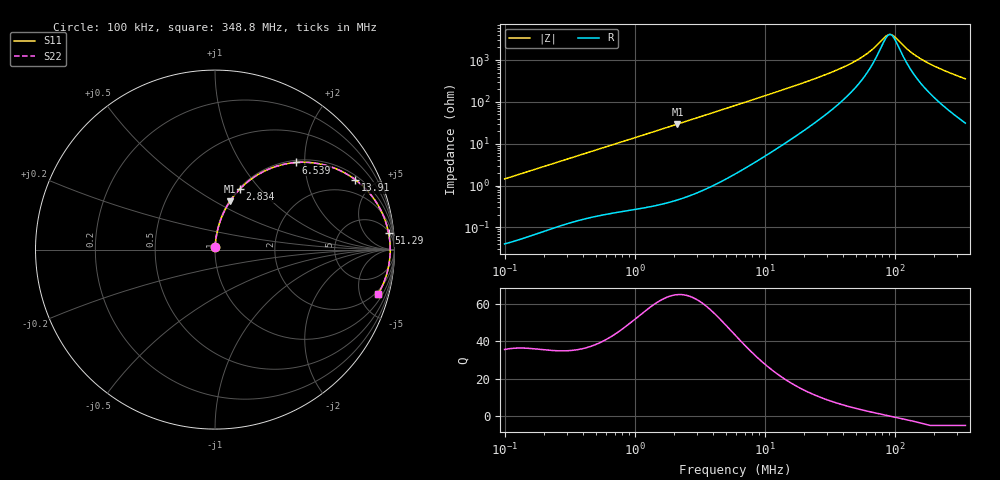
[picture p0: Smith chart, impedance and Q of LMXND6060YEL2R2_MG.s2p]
! LMXND6060YEL2R2_MG  S-PARAMETER MODEL  ( Standard Model )
! Model Generated by TAIYO YUDEN Corporation (http://www.ty-top.com)
! Version 1.0
! TAIYO YUDEN Control No. 20240226
! Copyright(c) 2024 TAIYO YUDEN CO.,LTD. All Rights Reserved.
! Product Description (link to TY-COMPAS)
! https://ds.yuden.co.jp/TYCOMPAS/or/detail?pn=LMXND6060YEL2R2NMG&u=M
! Products Name : Inductors
! Characteristics :
!  Inductance : 2.2 [uH] , SRF(min) : 60 [MHz] , DC Resistance(max) : 0.0286 [Ohm]
!  Rated Current : Saturation  6400 [mA] , Temp Rise  3600 [mA] (40 [degC])
!  Case Size : 6.0 x 6.0 / 0.236 x 0.236 [mm/inch] , Thickness : 4.5 / 0.177 [mm/inch]
!  (Conditions: Temperature = 25 [degC] , DC Bias Current = 0 [A])
! External Node Assignments :
!  1  o---GGG---o  2
! GND o---------o GND
! Frequency Range : 0.1MHz  -  348.750116MHz  [ 402 STEP ]
# MHz S RI R 50
! Freq[MHz].  S11 Real  S11 Imag  S21 Real  S21 Imag  S12 Real  S12 Imag  S22 Real  S22 Imag
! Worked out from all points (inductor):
!   401 points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, 100 kHz to 348.8 MHz, reference 50 ohm
!   read as one part in series: L = 2.29 uH near 104.2 kHz
!   highest Q = 65.1 at 2.13 MHz (marker M1), where L = 2.2 uH
!   self-resonance near 91.75 MHz
!   S11 on the Smith chart (normalised r, x): 100 kHz: 1.00, +0.03; 2.834 MHz: 1.01, +0.78; 6.539 MHz: 1.05, +1.81; 13.91 MHz: 1.19, +3.92; 51.29 MHz: 6, +19; 348.8 MHz: 1.62, -7.10
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0.1  0.00061 0.0144  0.9994 -0.0144  0.9994 -0.0144  0.00061 0.0144
0.392077  0.00455 0.0549  0.9954 -0.0549  0.9954 -0.0549  0.00455 0.0549
0.816954  0.0151 0.1116  0.9849 -0.1116  0.9849 -0.1116  0.0151 0.1116
1.537242  0.0463 0.2021  0.9537 -0.2021  0.9537 -0.2021  0.0463 0.2021
2.13031  0.0833 0.2687  0.9167 -0.2687  0.9167 -0.2687  0.0833 0.2687
2.834203  0.137 0.336  0.863 -0.336  0.863 -0.336  0.137 0.336
4.008554  0.2391 0.4176  0.7609 -0.4176  0.7609 -0.4176  0.2391 0.4176
5.905507  0.4033 0.4792  0.5967 -0.4792  0.5967 -0.4792  0.4033 0.4792
6.539411  0.4525 0.4855  0.5475 -0.4855  0.5475 -0.4855  0.4525 0.4855
9.249015  0.6204 0.4689  0.3796 -0.4689  0.3796 -0.4689  0.6204 0.4689
13.90661  0.7826 0.3886  0.2174 -0.3886  0.2174 -0.3886  0.7826 0.3886
23.15412  0.9022 0.258  0.0978 -0.258  0.0978 -0.258  0.9022 0.258
36.26324  0.9504 0.1564  0.0496 -0.1564  0.0496 -0.1564  0.9504 0.1564
51.28891  0.9674 0.0917  0.0326 -0.0917  0.0326 -0.0917  0.9674 0.0917
64.18634  0.9731 0.0547  0.0269 -0.0547  0.0269 -0.0547  0.9731 0.0547
83.67088  0.976 0.0139  0.024 -0.0139  0.024 -0.0139  0.976 0.0139
90.78195  0.9762 0.00159  0.0238 -0.00159  0.0238 -0.00159  0.9762 0.00159
98.49737  0.9761 -0.0107  0.0239 0.0107  0.0239 0.0107  0.9761 -0.0107
128.3974  0.9735 -0.0514  0.0265 0.0514  0.0265 0.0514  0.9735 -0.0514
163.9954  0.9675 -0.0916  0.0325 0.0916  0.0325 0.0916  0.9675 -0.0916
231.9469  0.9505 -0.1563  0.0495 0.1563  0.0495 0.1563  0.9505 -0.1563
348.7501  0.9086 -0.2478  0.0914 0.2478  0.0914 0.2478  0.9086 -0.2478
